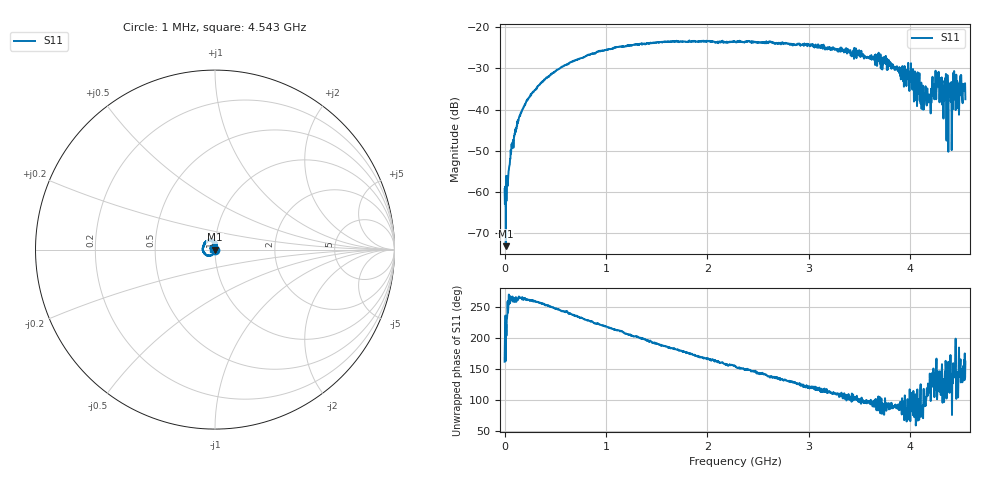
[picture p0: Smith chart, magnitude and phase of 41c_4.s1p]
# HZ S RI R 50
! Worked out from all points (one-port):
!   1515 points, 1 MHz to 4.543 GHz, reference 50 ohm
!   lowest |S11| = -73.3 dB at 13 MHz (marker M1), VSWR 1.00, Z = 50 + j0.00637 ohm
!   |S11| at or under -10 dB: start of sweep to end of sweep
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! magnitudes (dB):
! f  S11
! 1 MHz  -59.4
! 13 MHz  -73.3
! 31 MHz  -58.6
! 43 MHz  -54.7
! 82 MHz  -48.2
! 166 MHz  -40.5
! 343 MHz  -34.0
! 571 MHz  -29.5
! 1.138 GHz  -24.6
! 1.705 GHz  -23.5
! 2.272 GHz  -23.4
! 2.842 GHz  -24.4
! 3.409 GHz  -25.5
! 3.754 GHz  -27.1
! 3.976 GHz  -30.6
! 4.024 GHz  -31.6
! 4.114 GHz  -35.0
! 4.192 GHz  -36.3
! 4.264 GHz  -31.1
! 4.288 GHz  -38.2
! 4.309 GHz  -32.2
! 4.378 GHz  -36.0
! 4.384 GHz  -36.9
! 4.393 GHz  -35.8
! 4.444 GHz  -31.8
! 4.468 GHz  -33.9
! 4.507 GHz  -36.2
! 4.543 GHz  -37.5
